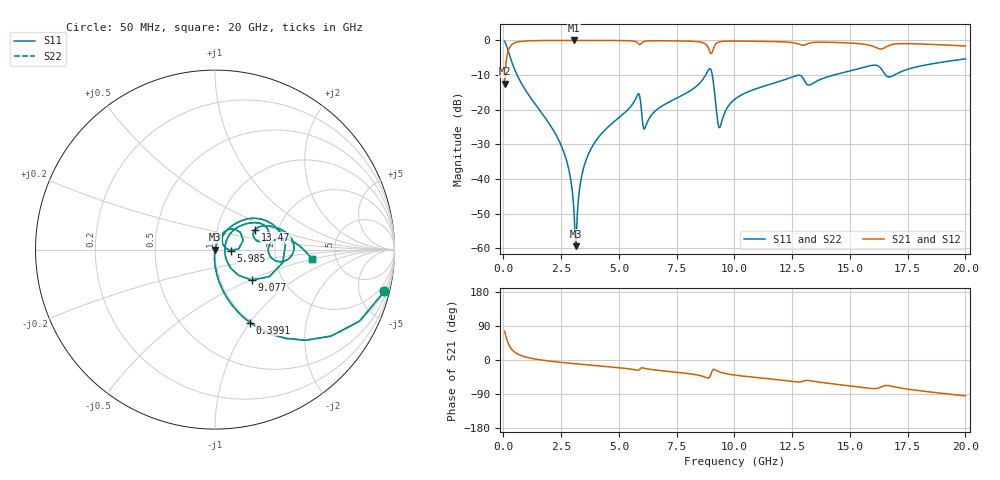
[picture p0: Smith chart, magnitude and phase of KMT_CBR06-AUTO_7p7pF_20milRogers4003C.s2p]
! Data measured by Modelithics Inc. support@modelithics.com 813-866-6335
! KEMET CBR06-AUTO 7.7pF, Pad Width= 0.851mm, Pad Length= 0.64mm, Pad Gap= 0.62mm, 20mil Rogers 4003C substrate Data, January 2022
# hz S ma R 50
! 2 Port Network Data from SP1.SP block
! freq  magS11  angS11  magS21  angS21  magS12  angS12  magS22  angS22
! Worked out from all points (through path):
!   401 points, 50 MHz to 20 GHz, reference 50 ohm
!   highest |S21| = -0.01 dB at 3.042 GHz (marker M1); lowest = -12.5 dB at 50 MHz (marker M2)
!   group delay of S21, straight-line fit = 14.4 ps
!   lowest |S11| = -59.4 dB at 3.142 GHz (marker M3), VSWR 1.00, Z = 50.1 + j0.0414 ohm
!   |S11| at or under -10 dB: 593.9 MHz to 8.751 GHz (8.157 GHz wide, 175 % of centre); 9.041 GHz to 14.29 GHz (5.248 GHz wide, 45 % of centre); 16.55 GHz to 16.92 GHz (371.5 MHz wide, 2.22 % of centre)
!   |S22| runs from -59.4 to -0.3 dB; largest |S21 - S12| = 0
!   S11 on the Smith chart (normalised r, x): 50 MHz: 0.98, -8.11; 399.1 MHz: 0.98, -1.00; 5.985 GHz: 1.19, -0.01; 9.077 GHz: 1.41, -0.51; 13.47 GHz: 1.52, +0.36; 20 GHz: 3.29, -0.49
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5e7  0.9715 -13.9  0.2369 76.1  0.2369 76.1  0.9715 -13.9
3.99125e8  0.4512 -64.4  0.8918 25.5  0.8918 25.5  0.4512 -64.4
2.54375e9  0.02819 -94.9  0.9987 -6.5  0.9987 -6.5  0.02819 -94.9
2.843e9  0.01311 -94.6  0.9989 -8.4  0.9989 -8.4  0.01311 -94.6
3.0425e9  0.00395 -86.5  0.999 -9.5  0.999 -9.5  0.00395 -86.5
3.14225e9  0.001077 22.6  0.999 -10.1  0.999 -10.1  0.001077 22.6
3.391625e9  0.01126 73.7  0.9989 -11.5  0.9989 -11.5  0.01126 73.7
4.33925e9  0.04886 71.9  0.9974 -16.7  0.9974 -16.7  0.04886 71.9
5.785625e9  0.1596 45.0  0.9393 -27.2  0.9393 -27.2  0.1596 45.0
5.985125e9  0.08808 -3.3  0.9153 -20.6  0.9153 -20.6  0.08808 -3.3
6.13475e9  0.05502 40.9  0.9738 -22.4  0.9738 -22.4  0.05502 40.9
6.73325e9  0.1058 60.0  0.9897 -27.5  0.9897 -27.5  0.1058 60.0
8.678375e9  0.2883 37.1  0.9143 -44.1  0.9143 -44.1  0.2883 37.1
9.077375e9  0.2657 -39.6  0.7404 -24.9  0.7404 -24.9  0.2657 -39.6
9.376625e9  0.05603 10.8  0.9578 -31.9  0.9578 -31.9  0.05603 10.8
1.0025e10  0.1425 46.4  0.9803 -39.9  0.9803 -39.9  0.1425 46.4
1.271825e10  0.3133 22.9  0.9012 -58.0  0.9012 -58.0  0.3133 22.9
1.336662e10  0.2374 24.6  0.9311 -55.5  0.9311 -55.5  0.2374 24.6
1.346638e10  0.2484 26.4  0.9382 -56.6  0.9382 -56.6  0.2484 26.4
1.601e10  0.4392 3.8  0.8207 -75.6  0.8207 -75.6  0.4392 3.8
1.670825e10  0.2967 0.1  0.8505 -68.1  0.8505 -68.1  0.2967 0.1
2e10  0.542 -5.6  0.8312 -94.7  0.8312 -94.7  0.542 -5.6
